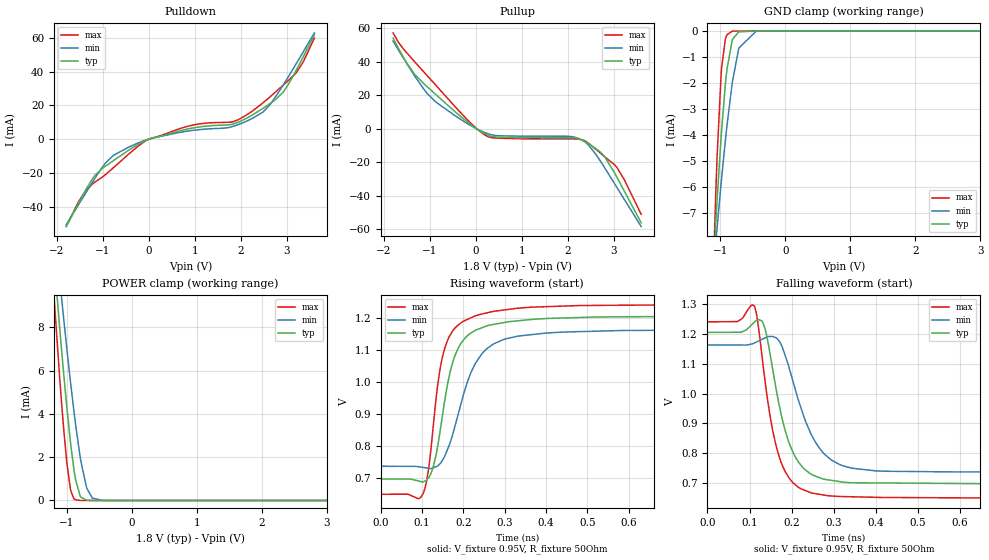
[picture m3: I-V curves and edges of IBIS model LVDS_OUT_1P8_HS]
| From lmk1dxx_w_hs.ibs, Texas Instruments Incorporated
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|   LVDS_OUT_1P8_HS Model
[Model]   LVDS_OUT_1P8_HS
Model_type   Output
Polarity   Non-Inverting
Vmeas = 0.95
Vref = 0.95
Cref = 2pF
Rref = 50
|   typ   min   max
C_comp   0.89pF   0.82pF   0.98pF
[Rac]   50   NA   NA
[Cac]   2p   NA   NA
[Voltage Range]   1.8   1.71   1.89
[Temperature Range]   45   150   -40
[Pullup Reference]   1.8   1.71   1.89
[Pulldown Reference]   0   0   0
[Power Clamp Reference]   1.8   1.71   1.89
[GND Clamp Reference]   0   0   0
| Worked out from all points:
|   slope of the pulldown table from 0 to 0.27 V, typ, clamps not added: 143 ohm
|   slope of the pullup table from 0 to 0.27 V, typ, clamps not added: 64.3 ohm
|   GND clamp passes 1 mA (typ) near -0.87 V on its own axis
|   POWER clamp passes 1 mA (typ) near -0.87 V on its own axis
|   falling waveform, V_fixture 0.95V, R_fixture 50Ohm: 20-80 % time 53.1ps typ, 68.9ps min, 46.2ps max; typ from 1.21 V to 0.695 V
|   rising waveform, V_fixture 0.95V, R_fixture 50Ohm: 20-80 % time 49.1ps typ, 68.7ps min, 39.7ps max; typ from 0.696 V to 1.2 V
[Pulldown]
|   Voltage   I(typ)   I(min)   I(max)
-1.8V     -51.74mA   -50.56mA   -51.58mA
-1.37V    -29.76mA   -31.62mA   -30.34mA
-1.169V   -21.22mA   -22.85mA   -25.27mA
-769.7mV  -12.66mA   -9.536mA   -16.82mA
-1.26mV   -17.91uA   -15.85uA   -21.46uA
974mV     6.67mA     5.239mA    8.401mA
1.85V     9.089mA    7.701mA    10.46mA
2.489V    18.37mA    16.18mA    21.62mA
2.918V    27.69mA    31.85mA    31.83mA
3.216V    41.28mA    45.12mA    39.62mA
3.362V    48.92mA    51.83mA    45.91mA
3.6V      61.74mA    62.89mA    59.79mA
[GND Clamp]
|   Voltage   I(typ)   I(min)   I(max)
-1.8V     -47.22mA   -32.28mA   -90.43mA
-1.103V   -8.782mA   -9.069mA   -8.722mA
-1.072V   -7.372mA   -8.153mA   -6.225mA
-1.053V   -6.556mA   -7.61mA    -4.893mA
-988.9mV  -4.055mA   -5.855mA   -1.636mA
-982.4mV  -3.827mA   -5.684mA   -1.42mA
-922.5mV  -2.008mA   -4.177mA   -294.7uA
-899.8mV  -1.477mA   -3.648mA   -144.9uA
-818.3mV  -346uA     -1.998mA   -5.222uA
-717.3mV  -29.3uA    -659.5uA   -36.6nA
-450mV    -2.385nA   -3.724uA   -4.984pA
3.6V      0A         0A         0A
[Pullup]
|   Voltage   I(typ)   I(min)   I(max)
-1.8V     53.97mA    52.25mA    57.15mA
-1.69V    48.28mA    47.24mA    51.76mA
-1.34V    32.7mA     31.86mA    40.24mA
-1.062V   25.11mA    21.13mA    31.75mA
-450mV    10.1mA     7.73mA     13.09mA
222.8mV   -3.388mA   -2.569mA   -4.173mA
498.8mV   -5.01mA    -4.202mA   -5.661mA
2.08V     -5.4mA     -4.715mA   -6.145mA
2.395V    -7.93mA    -8.34mA    -7.606mA
2.732V    -14.51mA   -20.15mA   -15.05mA
3.069V    -28.85mA   -34.97mA   -22.98mA
3.6V      -56.18mA   -58.39mA   -51.09mA
[POWER Clamp]
|   Voltage   I(typ)   I(min)   I(max)
-1.8V     35.35mA    33.02mA    38.41mA
-1.235V   12.58mA    14.14mA    11.07mA
-1.108V   7.901mA    10.18mA    5.58mA
-1.068V   6.535mA    8.999mA    4.045mA
-1V       4.324mA    7.032mA    1.764mA
-945.7mV  2.747mA    5.536mA    547.3uA
-890.1mV  1.424mA    4.11mA     81.35uA
-863.6mV  938uA      3.477mA    28.21uA
-793.4mV  199.1uA    1.989mA    1.463uA
-694.6mV  11.18uA    577.1uA    13.82nA
-607.7mV  708.9nA    109.9uA    193pA
3.6V      0A         0A         0A
[Ramp]
R_load = 50
|   typ   min   max
dV/dt_r   0.305338/4.90956e-11   0.25614/6.80011e-11   0.355006/3.97427e-11
dV/dt_f   0.30566/5.30348e-11   0.256826/6.88404e-11   0.355182/4.62238e-11
[Falling Waveform]
V_fixture = 0.95V
V_fixture_min = 0.95V
V_fixture_max = 0.95V
R_fixture = 50Ohm
C_fixture = 0F
|   Time   V(typ)   V(min)   V(max)
0s        1.205V     1.163V     1.24V
71.55ps   1.205V     1.162V     1.241V
110.9ps   1.238V     1.169V     1.294V
136.5ps   1.219V     1.186V     1.048V
155.6ps   1.078V     1.191V     873.6mV
174.6ps   935.4mV    1.166V     772.5mV
216.3ps   771mV      978.1mV    686.5mV
285.2ps   711.6mV    788.8mV    658.3mV
583.6ps   699.1mV    737.8mV    651mV
5ns       695.3mV    734.6mV    648.1mV
[Rising Waveform]
V_fixture = 0.95V
V_fixture_min = 0.95V
V_fixture_max = 0.95V
R_fixture = 50Ohm
C_fixture = 0F
|   Time   V(typ)   V(min)   V(max)
0s        695.6mV    735.6mV    648.1mV
103.1ps   687mV      732mV      651mV
115.7ps   699.7mV    729.5mV    725.7mV
125.6ps   727.6mV    730.1mV    840.2mV
144ps     847.2mV    744.5mV    1.042V
174.6ps   1.061V     837.2mV    1.159V
229.3ps   1.161V     1.058V     1.206V
273.3ps   1.179V     1.118V     1.22V
329.9ps   1.19V      1.142V     1.229V
5ns       1.204V     1.163V     1.24V
